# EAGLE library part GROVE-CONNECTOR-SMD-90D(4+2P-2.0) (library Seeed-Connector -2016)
320110032
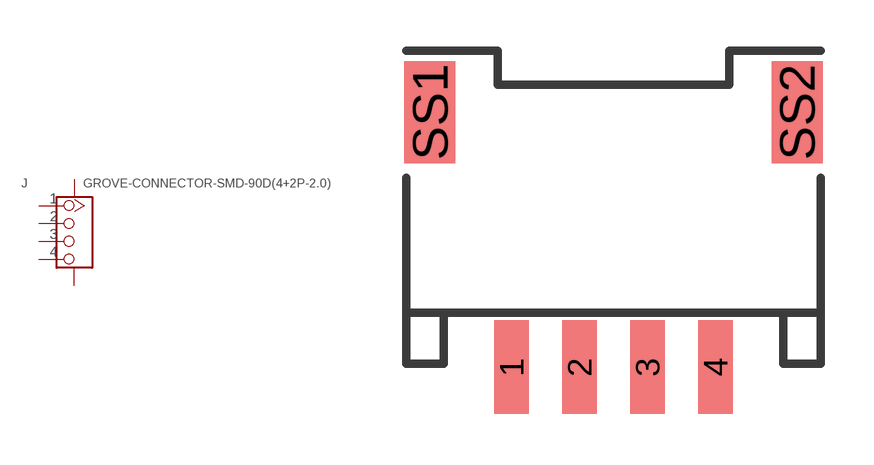
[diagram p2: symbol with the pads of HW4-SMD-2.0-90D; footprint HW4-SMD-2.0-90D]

Designator prefix J

## GROVE-CONNECTOR-SMD-90D(4+2P-2.0) (VALUE: 4P-SMD-2.0-90D)  [HW4-SMD-2.0-90D]
1  1
2  2
3  3
4  4
SS1  SS1
SS2  SS2

## Footprint HW4-SMD-2.0-90D (pad centres in mm)
smd 1.01 x 2.74: 1 -3,-0.1; 2 -1,-0.1; 3 1,-0.1; 4 3,-0.1
smd 1.5 x 3: SS1 -5.4,7.4; SS2 5.4,7.4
